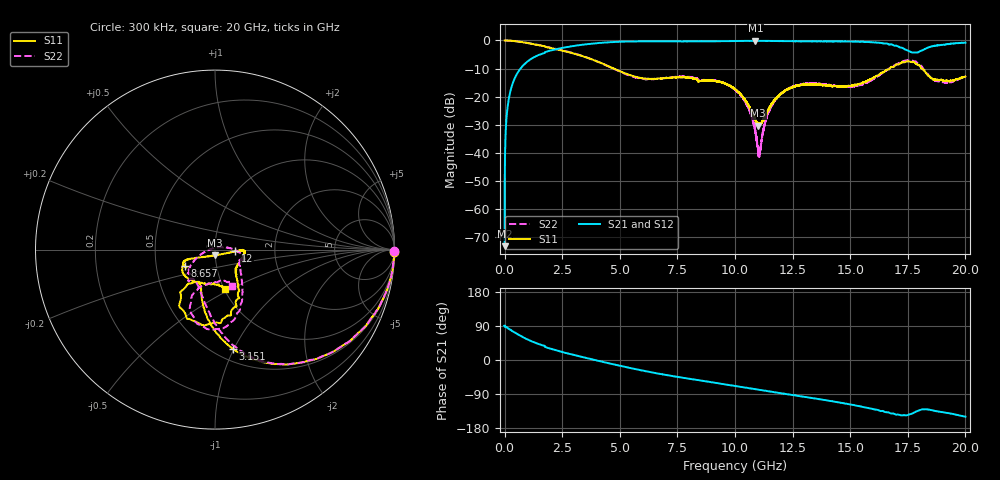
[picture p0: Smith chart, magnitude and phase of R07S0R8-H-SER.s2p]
!{R07S0R8}
!Johanson Technology Inc.
!www.johansontechnology.com
!Test Board Conditions:
!Substrate Type  RO4350B
!Substrate Thickness  10 mil
!Substrate Dk  3.66
!TL Type: GCPW
!TL Trace Width  21 mil
!TL Gap  20 mil
!Electrode orientation  Horizontal
!DUT TOPOLOGY	SERIES
!Mounting Pad LxW  16x21 mil
! Created Fri Feb  5 23:07:00 2021
# hz S ma R 50
! 2 Port Network Data from SP1.SP block
! freq  magS11  angS11  magS21  angS21  magS12  angS12  magS22  angS22
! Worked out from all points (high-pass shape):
!   20001 points, 300 kHz to 20 GHz, reference 50 ohm
!   highest |S21| = -0.13 dB at 10.88 GHz (marker M1); lowest = -73.1 dB at 300 kHz (marker M2)
!   |S21| within 3 dB of the highest: 2.224 GHz to 17.36 GHz (15.14 GHz wide, 155 % of centre); 18.22 GHz to end of sweep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
!   lowest |S11| = -30.3 dB at 11.01 GHz (marker M3), VSWR 1.06, Z = 49.9 - j3.07 ohm
!   |S11| at or under -10 dB: 4.746 GHz to 16.71 GHz (11.97 GHz wide, 112 % of centre); 18.1 GHz to end of sweep
!   |S22| runs from -41.8 to 0.0 dB; largest |S21 - S12| = 0.016
!   S11 on the Smith chart (normalised r, x): 300 kHz: open; 3.151 GHz: 0.61, -0.99; 8.657 GHz: 0.70, -0.13; 12 GHz: 1.25, -0.02; 20 GHz: 1.01, -0.47
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300000  0.9994 -0.6  0.0002205 90.1  0.0002231 70.9  1 -0.5
1.013e8  0.9963 -4.1  0.05119 85.7  0.05123 85.8  0.9967 -4.0
1.333e8  0.9975 -5.4  0.06731 84.3  0.06735 84.4  0.9975 -5.4
4.893e8  0.9686 -18.9  0.2342 70.7  0.2338 70.6  0.9697 -18.7
1.5053e9  0.8213 -48.5  0.5563 41.6  0.5563 41.5  0.8281 -47.6
3.1513e9  0.5618 -79.6  0.8167 11.2  0.8153 11.2  0.5692 -77.1
3.3343e9  0.5336 -82.5  0.8354 8.4  0.8342 8.4  0.5386 -79.7
6.6673e9  0.2095 -121.0  0.9683 -35.8  0.9676 -35.8  0.2088 -128.8
8.6573e9  0.1921 -152.0  0.9667 -55.5  0.9662 -55.5  0.1988 -137.9
1.00003e10  0.1365 -158.9  0.9761 -68.5  0.9775 -68.5  0.1334 -152.2
1.05453e10  0.07529 -146.8  0.9834 -73.7  0.9825 -73.7  0.06762 -165.4
1.08823e10  0.03895 -116.8  0.9857 -77.0  0.9839 -76.9  0.02547 173.7
1.10093e10  0.03071 -90.6  0.9835 -78.2  0.9836 -78.2  0.0101 137.7
1.14803e10  0.06308 -19.6  0.9822 -82.8  0.9804 -82.8  0.05607 13.5
1.19973e10  0.1127 -4.6  0.9751 -87.7  0.9762 -87.8  0.1126 -1.2
1.33343e10  0.1675 -7.1  0.9631 -100.2  0.9641 -100.2  0.1729 -18.3
1.53293e10  0.1664 -46.4  0.9509 -121.1  0.9535 -121.2  0.1567 -29.8
1.66673e10  0.3042 -66.1  0.852 -138.5  0.857 -139.1  0.3129 -61.0
1.74703e10  0.4242 -97.2  0.6678 -145.6  0.6707 -145.4  0.4418 -87.1
1.79843e10  0.3629 -123.1  0.6291 -133.0  0.631 -132.7  0.378 -110.6
1.87423e10  0.1991 -111.1  0.8115 -135.1  0.814 -135.2  0.1908 -98.8
2e10  0.2281 -75.8  0.913 -149.7  0.9105 -149.6  0.2247 -65.1
